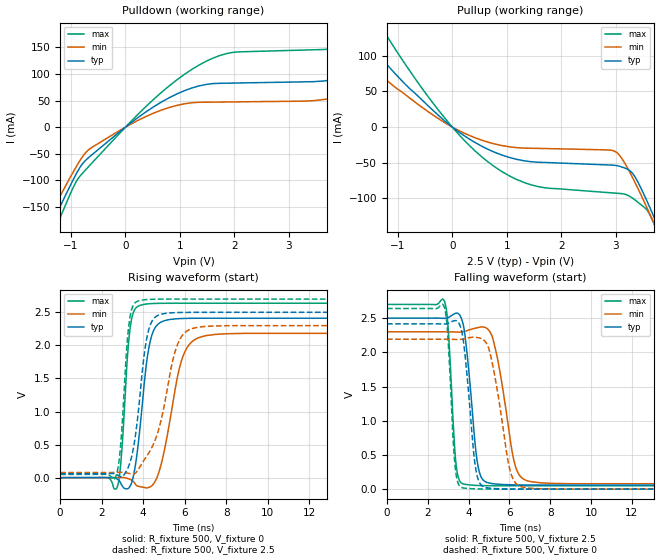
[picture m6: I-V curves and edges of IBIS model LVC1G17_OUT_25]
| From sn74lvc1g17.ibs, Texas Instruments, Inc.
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[Model]   LVC1G17_OUT_25
Model_type  Output
Vref =   0
Rref =   500
Cref =   30p
Vmeas =   1.25
| variable   typ   min   max
C_comp   9.69pF   6.16pF   13.53pF
| C_pullup   9.65pF   6.16pF   11.31pF
| C_pulldown   9.72pF   6.35pF   13.53pF
[Temperature Range]   40   100   -40
| Ambient temperature   25   85   -40
[Voltage range]   2.5   2.3   2.7
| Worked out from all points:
|   slope of the pulldown table from 0 to 0.375 V, typ, clamps not added: 13.1 ohm
|   slope of the pullup table from 0 to 0.375 V, typ, clamps not added: 19 ohm
|   rising waveform, R_fixture 500, V_fixture 0: 20-80 % time 504ps typ, 789ps min, 321ps max; typ from 0 V to 2.41 V
|   falling waveform, R_fixture 500, V_fixture 2.5: 20-80 % time 445ps typ, 700ps min, 286ps max; typ from 2.5 V to 0.06 V
|   rising waveform, R_fixture 500, V_fixture 2.5: 20-80 % time 535ps typ, 978ps min, 328ps max; typ from 0.06 V to 2.5 V
|   falling waveform, R_fixture 500, V_fixture 0: 20-80 % time 432ps typ, 695ps min, 276ps max; typ from 2.42 V to 0 V
[Pulldown]
| LVC1G17_OUT_25
|   Voltage   I(typ)   I(min)   I(max)
-5.5V     -1.065A    -962.2mA   -1.199A
-1.53V    -221.1mA   -193.8mA   -251.2mA
-1.17V    -142.7mA   -123.7mA   -162.8mA
-670mV    -56.67mA   -41.91mA   -73.36mA
520mV     38.43mA    26.46mA    52.49mA
1.485V    80.34mA    46.87mA    124mA
3.84V     90.07mA    55.63mA    147.9mA
5.34V     157.5mA    105.9mA    231.4mA
5.91V     188.7mA    52.63mA    282.8mA
6.525V    93.57mA    53.14mA    298.9mA
7.56V     94.12mA    54.12mA    160.7mA
11V       99.65mA    57.57mA    168.9mA
[Pullup]
| LVC1G17_OUT_25
|   Voltage   I(typ)   I(min)   I(max)
-5.5V     533.4mA    418.6mA    746.4mA
-2.34V    192.7mA    147.4mA    275.6mA
-1.735V   134.9mA    102mA      194.6mA
-1.32V    97.81mA    73.23mA    142.1mA
-135mV    8.418mA    6.055mA    12.49mA
750mV     -34.38mA   -23.05mA   -54.11mA
1.57V     -49.22mA   -29.81mA   -83.34mA
2.995V    -53.63mA   -34.3mA    -92.61mA
3.315V    -65.3mA    -71.46mA   -99.87mA
3.565V    -101.9mA   -111.4mA   -115.4mA
3.75V     -134.3mA   -142.6mA   -143.5mA
11V       -1.614A    -1.516A    -1.761A
[Ramp]
| LVC1G17_OUT_25
| variable   typ   min   max
dV/dt_r   1.55/5.43E-10   1.40/8.48E-10   1.69/3.46E-10
dV/dt_f   1.51/4.63E-10   1.38/7.31E-10   1.64/2.97E-10
R_load = 500
[Rising Waveform]
| LVC1G17_OUT_25
R_fixture =   500
C_fixture =   0
L_fixture =   0
V_fixture =   0
V_fixture_min = 0
V_fixture_max = 0
|   Time   V(typ)   V(min)   V(max)
0s        123.5pV    5.747nV    2.756nV
2.74ns    -19.42mV   3.094mV    -149.4mV
2.945ns   -100.4mV   3.82mV     307.5mV
3.365ns   -131.4mV   -24.81mV   2.245V
3.855ns   782mV      -136.9mV   2.605V
4.2ns     1.822V     -153.2mV   2.627V
4.535ns   2.245V     -77.97mV   2.634V
5.845ns   2.406V     1.768V     2.637V
6.72ns    2.41V      2.122V     2.637V
24.5ns    2.411V     2.183V     2.637V
[Falling Waveform]
| LVC1G17_OUT_25
R_fixture =   500
C_fixture =   0
L_fixture =   0
V_fixture =   2.5
V_fixture_min = 2.3
V_fixture_max = 2.7
|   Time   V(typ)   V(min)   V(max)
0s        2.5V       2.3V       2.7V
2.82ns    2.496V     2.3V       2.743V
3ns       2.508V     2.3V       2.327V
3.365ns   2.572V     2.297V     414mV
3.695ns   2.451V     2.299V     80.74mV
4.415ns   412.6mV    2.358V     54.46mV
4.89ns    99.46mV    2.351V     51.03mV
6.245ns   63.04mV    385.8mV    49.49mV
6.81ns    61.3mV     129.4mV    49.43mV
24.5ns    60.11mV    77.11mV    49.35mV
[Rising Waveform]
| LVC1G17_OUT_25
R_fixture =   500
C_fixture =   0
L_fixture =   0
V_fixture =   2.5
V_fixture_min = 2.3
V_fixture_max = 2.7
|   Time   V(typ)   V(min)   V(max)
0s        60.06mV    77.04mV    49.31mV
2.67ns    52.71mV    79.41mV    9.173mV
2.905ns   15.08mV    80.48mV    461.6mV
3.32ns    187.9mV    63.71mV    2.33V
3.74ns    924.5mV    112mV      2.669V
4.09ns    1.952V     289.2mV    2.69V
4.405ns   2.355V     449.5mV    2.696V
5.59ns    2.495V     1.958V     2.7V
6.335ns   2.499V     2.252V     2.7V
24.5ns    2.5V       2.3V       2.7V
[Falling Waveform]
| LVC1G17_OUT_25
R_fixture =   500
C_fixture =   0
L_fixture =   0
V_fixture =   0
V_fixture_min = 0
V_fixture_max = 0
|   Time   V(typ)   V(min)   V(max)
0s        2.416V     2.191V     2.64V
2.79ns    2.413V     2.192V     2.673V
2.97ns    2.421V     2.191V     2.284V
3.335ns   2.464V     2.189V     335.9mV
3.675ns   2.287V     2.191V     21.65mV
4.32ns    347.1mV    2.22V      4.501mV
4.775ns   29.82mV    2.169V     1.538mV
6.01ns    2.204mV    296.6mV    183.1uV
6.535ns   910.5uV    39.37mV    119.3uV
24.5ns    42.92uV    60.76uV    35.64uV
